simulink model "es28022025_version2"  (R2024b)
settings: Solver=ode4  StartTime=0.0  StopTime=5  FixedStep=0.005  RelTol=1e-3
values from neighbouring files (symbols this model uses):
  a = 0.5    [scriptsimulink28022025.m]
  xzero = 1    [scriptsimulink28022025.m]
  yzero = 2    [scriptsimulink28022025.m]
  yzerodot = -1    [scriptsimulink28022025.m]

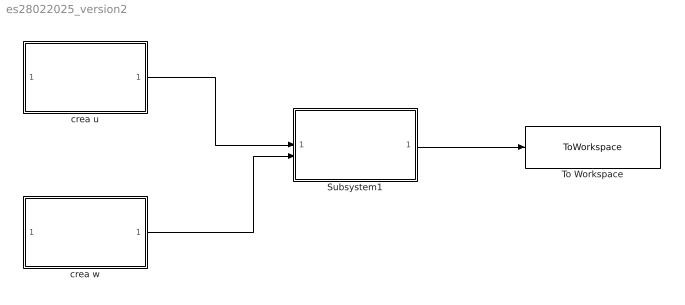
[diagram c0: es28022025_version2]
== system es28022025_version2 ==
  Subsystem1 : Subsystem
  To Workspace : ToWorkspace  VariableName=y  SaveFormat=Timeseries  SampleTime=-1
  crea u : Subsystem
  crea w : Subsystem
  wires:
  crea u/1(u) -> Subsystem1/1(u)
  crea w/1(w) -> Subsystem1/2(w)
  Subsystem1/1(y) -> To Workspace/1

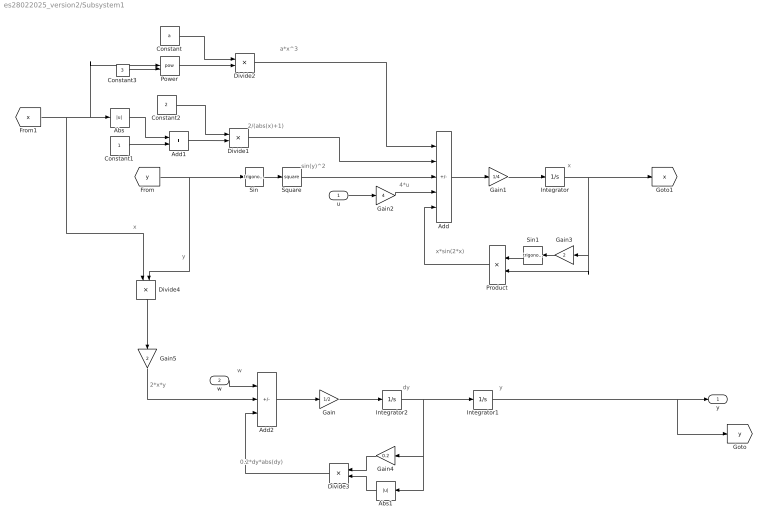
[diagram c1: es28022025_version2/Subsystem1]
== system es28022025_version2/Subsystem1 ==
  note: x
  note: y
  note: 0.2*dy*abs(dy)
  note: w
  note: 2*x*y
  note: a*x^3
  note: 2/(abs(x)+1)
  note: sin(y)^2
  note: 4*u
  note: x*sin(2*x)
  note: y
  note: dy
  note: x
  u : Inport
  w : Inport  Port=2
  Abs : Abs
  Abs1 : Abs
  Add : Sum  Inputs=---++
  Add1 : Sum
  Add2 : Sum  Inputs=+--
  Constant : Constant  Value=a
  Constant1 : Constant
  Constant2 : Constant  Value=2
  Constant3 : Constant  Value=3
  Divide1 : Product  Inputs=*/
  Divide2 : Product
  Divide3 : Product
  Divide4 : Product
  Gain : Gain  Gain=1/2
  Gain1 : Gain  Gain=1/4
  Gain2 : Gain  Gain=4
  Gain3 : Gain  Gain=2
  Gain4 : Gain  Gain=0.2
  Gain5 : Gain  Gain=2
  Integrator : Integrator  InitialCondition=xzero
  Integrator1 : Integrator  InitialCondition=yzero
  Integrator2 : Integrator  InitialCondition=yzerodot
  Power : Math  Operator=pow  SignedPower=on
  Product : Product
  Sin : Trigonometry
  Sin1 : Trigonometry
  Square : Math  Operator=square  SignedPower=on
  y : Outport  VectorParamsAs1DForOutWhenUnconnected=off
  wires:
  Integrator/1 -> Product/2, Gain3/1, [x]
  Gain1/1 -> Integrator/1
  Add/1 -> Gain1/1
  u/1 -> Gain2/1
  Gain3/1 -> Sin1/1
  Sin1/1 -> Product/1
  Gain2/1 -> Add/4
  Product/1 -> Add/5
  Sin/1 -> Square/1
  Square/1 -> Add/3
  [y] -> Divide4/2, Sin/1
  Constant1/1 -> Add1/2
  [x] -> Divide4/1, Power/1, Abs/1
  Abs/1 -> Add1/1
  Add1/1 -> Divide1/2
  Constant2/1 -> Divide1/1
  Divide1/1 -> Add/2
  Constant3/1 -> Power/2
  Power/1 -> Divide2/2
  Constant/1 -> Divide2/1
  Divide2/1 -> Add/1
  Integrator1/1 -> [y], y/1
  Integrator2/1 -> Abs1/1, Gain4/1, Integrator1/1
  Gain/1 -> Integrator2/1
  Add2/1 -> Gain/1
  w/1 -> Add2/1
  Gain4/1 -> Divide3/1
  Abs1/1 -> Divide3/2
  Divide3/1 -> Add2/3
  Gain5/1 -> Add2/2
  Divide4/1 -> Gain5/1

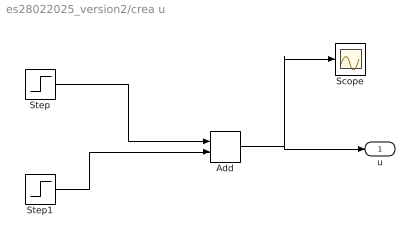
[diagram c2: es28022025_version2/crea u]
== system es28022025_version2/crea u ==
  Add : Sum
  Scope : Scope
  Step : Step  Time=2  Before=2  After=6  SampleTime=0
  Step1 : Step  Time=3  After=-4  SampleTime=0
  u : Outport  VectorParamsAs1DForOutWhenUnconnected=off
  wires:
  Step/1 -> Add/1
  Step1/1 -> Add/2
  Add/1 -> Scope/1, u/1

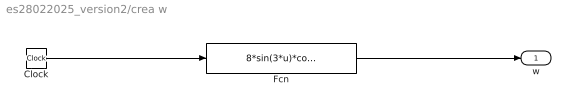
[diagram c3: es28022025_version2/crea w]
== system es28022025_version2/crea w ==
  Clock : Clock
  Fcn : Fcn  Expr=8*sin(3*u)*cos(10*u+0.1)
  w : Outport  VectorParamsAs1DForOutWhenUnconnected=off
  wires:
  Clock/1 -> Fcn/1
  Fcn/1 -> w/1
